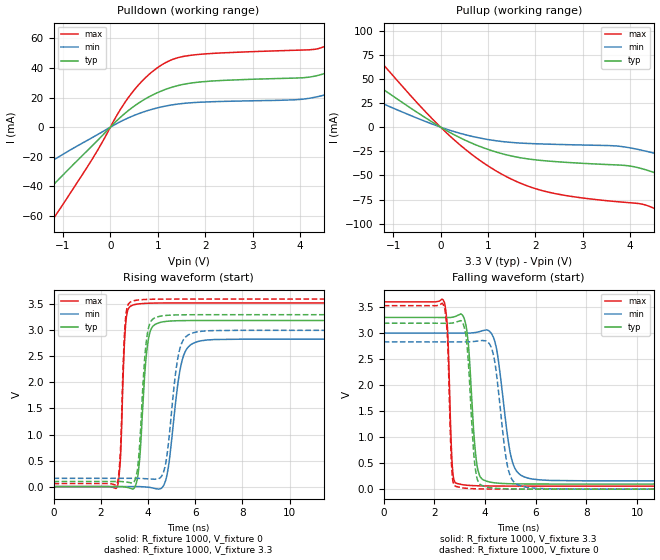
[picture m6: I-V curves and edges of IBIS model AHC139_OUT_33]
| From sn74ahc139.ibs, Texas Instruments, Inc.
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[Model]   AHC139_OUT_33
Model_type  Output
Vref =   0
Rref =   1000
Cref =   50p
Vmeas =   1.65
| variable   typ   min   max
C_comp   2.48pF   1.84pF   3.22pF
| C_pullup   2.61pF   1.84pF   3.22pF
| C_pulldown   2.35pF   1.90pF   2.88pF
[Temperature Range]   40   100   -40
| Ambient temperature   25   85   -40
[Voltage range]   3.3   3   3.6
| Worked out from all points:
|   slope of the pulldown table from 0 to 0.495 V, typ, clamps not added: 35.3 ohm
|   slope of the pullup table from 0 to 0.495 V, typ, clamps not added: 38.2 ohm
|   rising waveform, R_fixture 1000, V_fixture 0: 20-80 % time 272ps typ, 449ps min, 163ps max; typ from 0 V to 3.19 V
|   falling waveform, R_fixture 1000, V_fixture 3.3: 20-80 % time 253ps typ, 446ps min, 137ps max; typ from 3.3 V to 0.098 V
|   rising waveform, R_fixture 1000, V_fixture 3.3: 20-80 % time 264ps typ, 412ps min, 160ps max; typ from 0.098 V to 3.3 V
|   falling waveform, R_fixture 1000, V_fixture 0: 20-80 % time 238ps typ, 403ps min, 131ps max; typ from 3.19 V to 0 V
[Pulldown]
| AHC139_OUT_33
|   Voltage   I(typ)   I(min)   I(max)
-5.5V     -169.6mA   -106.1mA   -213.5mA
-3.83V    -120.2mA   -73.54mA   -157.4mA
-2.135V   -69.06mA   -40.48mA   -100.8mA
-1.29V    -41.79mA   -23.97mA   -65.93mA
450mV     12.96mA    7.25mA     23.01mA
965mV     22.89mA    12.81mA    39.52mA
1.43V     28.14mA    15.63mA    46.99mA
4.38V     34.95mA    20.64mA    53.01mA
5.26V     47mA       29.64mA    70.03mA
6.305V    69.65mA    45.48mA    104mA
7.59V     104.9mA    69.49mA    156.3mA
11V       223.4mA    143.6mA    338.2mA
[Pullup]
| AHC139_OUT_33
|   Voltage   I(typ)   I(min)   I(max)
-5.5V     206.8mA    122mA      360.9mA
-4.63V    169.5mA    101.8mA    290.6mA
-3V       104.1mA    64.04mA    174.1mA
-1.92V    64.06mA    39.62mA    106.2mA
405mV     -10.85mA   -6.308mA   -18.2mA
1.335V    -27.98mA   -15.09mA   -49.85mA
2.215V    -34.88mA   -17.54mA   -66.59mA
4.32V     -44.01mA   -24.75mA   -80.54mA
5.315V    -63.19mA   -38.26mA   -106.1mA
6.925V    -103.2mA   -64.95mA   -156mA
9.095V    -163.5mA   -104.8mA   -226.6mA
11V       -219.9mA   -141.8mA   -291.3mA
[Ramp]
| AHC139_OUT_33
| variable   typ   min   max
dV/dt_r   1.94/2.80E-10   1.73/4.60E-10   2.14/1.72E-10
dV/dt_f   1.96/2.65E-10   1.74/4.62E-10   2.16/1.40E-10
R_load = 1000
[Rising Waveform]
| AHC139_OUT_33
R_fixture =   1000
C_fixture =   0
L_fixture =   0
V_fixture =   0
V_fixture_min = 0
V_fixture_max = 0
|   Time   V(typ)   V(min)   V(max)
0s        1.228nV    2.082nV    700.3pV
2.69ns    1.189mV    185uV      -4.76mV
2.835ns   1.016mV    311.5uV    543.5mV
3.07ns    -10.47mV   550.3uV    3.186V
3.485ns   32.42mV    1.047mV    3.499V
4.01ns    2.806V     -12.04mV   3.52V
4.605ns   3.161V     -15.46mV   3.525V
5.445ns   3.186V     2.418V     3.526V
6.27ns    3.188V     2.801V     3.526V
40ns      3.189V     2.83V      3.526V
[Falling Waveform]
| AHC139_OUT_33
R_fixture =   1000
C_fixture =   0
L_fixture =   0
V_fixture =   3.3
V_fixture_min = 3
V_fixture_max = 3.6
|   Time   V(typ)   V(min)   V(max)
0s        3.3V       3V         3.6V
2.385ns   3.299V     3V         3.6V
2.525ns   3.298V     3V         3.02V
2.725ns   3.305V     2.999V     337.4mV
3.11ns    3.344V     2.999V     86.62mV
3.695ns   424.5mV    3.017V     65.26mV
4.26ns    130.5mV    2.987V     60.65mV
5.07ns    103.4mV    541.6mV    58.99mV
5.875ns   99.15mV    194mV      58.6mV
40ns      97.8mV     159.3mV    58.46mV
[Rising Waveform]
| AHC139_OUT_33
R_fixture =   1000
C_fixture =   0
L_fixture =   0
V_fixture =   3.3
V_fixture_min = 3
V_fixture_max = 3.6
|   Time   V(typ)   V(min)   V(max)
0s        97.8mV     159.3mV    58.46mV
2.68ns    98.56mV    159.5mV    52.91mV
2.83ns    98.18mV    159.5mV    650.9mV
3.06ns    88.54mV    159.5mV    3.271V
3.455ns   129.3mV    159.3mV    3.573V
3.975ns   2.933V     150.2mV    3.594V
4.53ns    3.272V     174.6mV    3.599V
5.335ns   3.297V     2.617V     3.6V
6.095ns   3.3V       2.971V     3.6V
40ns      3.3V       3V         3.6V
[Falling Waveform]
| AHC139_OUT_33
R_fixture =   1000
C_fixture =   0
L_fixture =   0
V_fixture =   0
V_fixture_min = 0
V_fixture_max = 0
|   Time   V(typ)   V(min)   V(max)
0s        3.189V     2.83V      3.526V
2.37ns    3.188V     2.83V      3.528V
2.515ns   3.188V     2.83V      2.926V
2.715ns   3.194V     2.83V      214.7mV
3.08ns    3.223V     2.83V      27.46mV
3.635ns   335mV      2.842V     7.085mV
4.165ns   32.04mV    2.798V     2.459mV
4.925ns   5.954mV    362.1mV    656uV
5.665ns   1.605mV    33.4mV     205uV
40ns      -7.332nV   -15.89nV   -2.554nV
